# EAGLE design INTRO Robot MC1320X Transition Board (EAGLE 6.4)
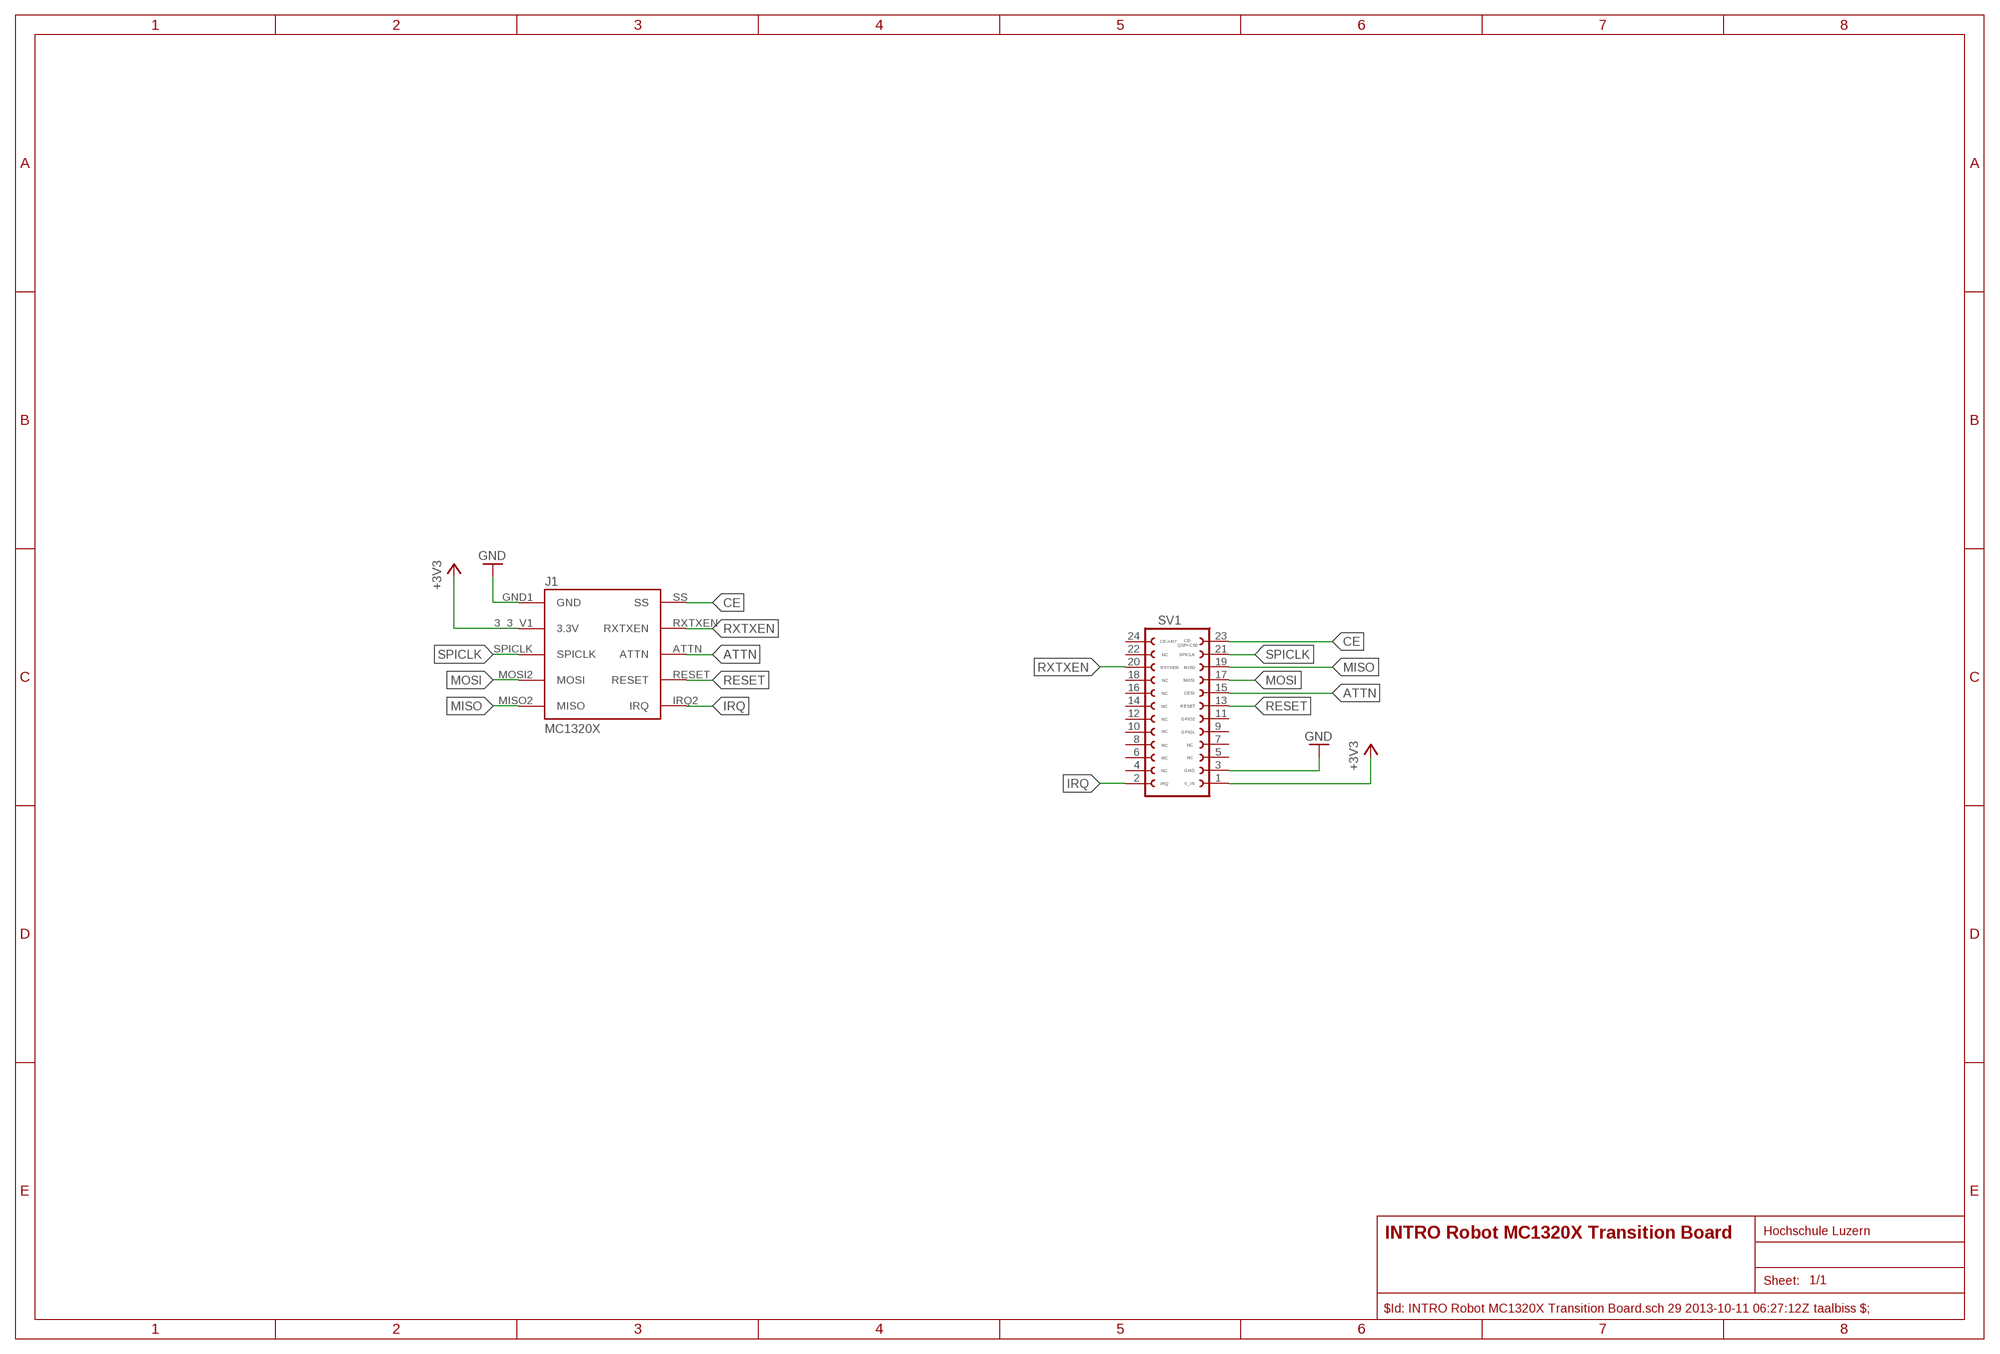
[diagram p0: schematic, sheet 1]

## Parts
J1  MC1320X  MC1320X_MOTHERBOARD  [MC1320X_MOTHERBOARD]
SV1  MC1320X  [FE12-2]

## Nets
+3V3: J1.3_3_V1(3.3V) SV1.1
ATTN: J1.ATTN SV1.15
CE: J1.SS SV1.23
GND: J1.GND1(GND) SV1.3
IRQ: J1.IRQ2(IRQ) SV1.2
MISO: J1.MISO2(MISO) SV1.19
MOSI: J1.MOSI2(MOSI) SV1.17
RESET: J1.RESET SV1.13
RXTXEN: J1.RXTXEN SV1.20
SPICLK: J1.SPICLK SV1.21
Unconnected: SV1.4 SV1.5 SV1.6 SV1.7 SV1.8 SV1.9 SV1.10 SV1.11 SV1.12 SV1.14 SV1.16 SV1.18 SV1.22 SV1.24

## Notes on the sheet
- $Id: INTRO Robot MC1320X Transition Board.sch 29 2013-10-11 06:27:12Z taalbiss $;

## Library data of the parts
J1 = MC1320X_Header_Motherboard:MC1320X_MOTHERBOARD
SV1 = Freescale MC1320x:MC1320X: Freescale MC1320x RF Daughter Board Connector

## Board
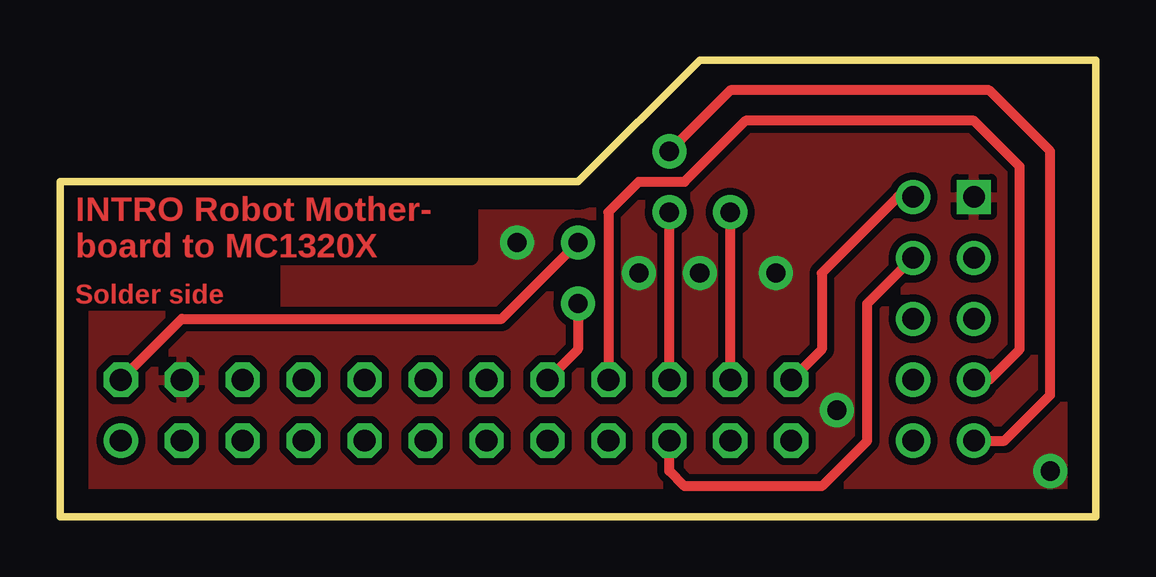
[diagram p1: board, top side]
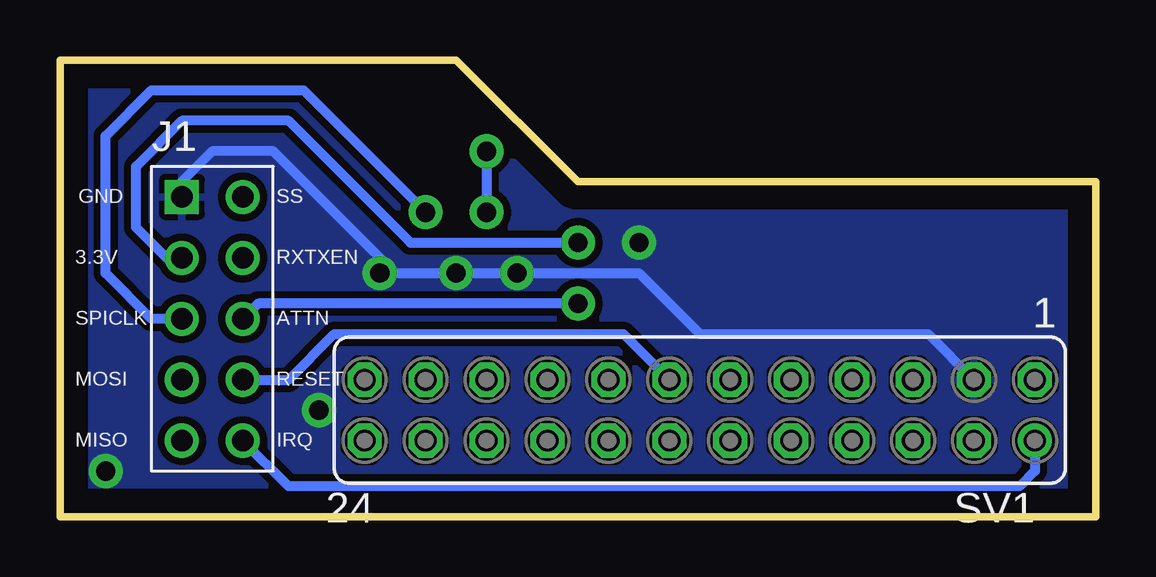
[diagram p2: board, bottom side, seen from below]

Size 43.18 x 19.05 mm. Coordinates in mm from the lower left corner, seen from the top.
Outline: 0,0 43.18,0 43.18,19.05 26.67,19.05 21.59,13.97 0,13.97 0,0
Copper layers (1*16): Top 0.035mm / dielectric 1.5mm / Bottom 0.035mm
Design rules "default": minimum track width 10mil, minimum drill 24mil, track to track 8mil, track to pad 8mil, pad to pad 8mil, via to via 8mil, smd to smd 8mil, copper to edge 40mil, drill to drill 8mil, minimum pad ring 10mil, minimum via ring 8mil, stop-mask expansion 4mil, vias tented up to drill 0mil, thermal gap 10mil
tRestrict: area 0,8.9 to 8.9,14; area 8.9,10.8 to 17.1,14

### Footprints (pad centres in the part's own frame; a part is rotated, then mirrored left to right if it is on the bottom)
MC1320X_MOTHERBOARD = drill 0.9 pad 1.422: 3_3_V1 -1.27,3.81; ATTN 1.27,1.27; IRQ2 1.27,-3.81; MISO2 -1.27,-3.81; MOSI2 -1.27,-1.27; RESET 1.27,-1.27; RXTXEN 1.27,3.81; SPICLK -1.27,1.27; SS 1.27,6.35 | drill 0.9 pad 1.422 square: GND1 -1.27,6.35
FE12-2 = drill 0.914 octagon: 1 -13.97,-1.27; 3 -11.43,-1.27; 4 -11.43,1.27; 5 -8.89,-1.27; 6 -8.89,1.27; 7 -6.35,-1.27; 8 -6.35,1.27; 9 -3.81,-1.27; 10 -3.81,1.27; 11 -1.27,-1.27; 12 -1.27,1.27; 13 1.27,-1.27; 14 1.27,1.27; 15 3.81,-1.27; 16 3.81,1.27; 17 6.35,-1.27; 18 6.35,1.27; 19 8.89,-1.27; 20 8.89,1.27; 21 11.43,-1.27; 22 11.43,1.27; 23 13.97,-1.27; 24 13.97,1.27 | drill 0.914: 2 -13.97,1.27

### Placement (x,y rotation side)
J1  36.83,6.99 0 bottom
SV1  16.51,4.45 180 bottom

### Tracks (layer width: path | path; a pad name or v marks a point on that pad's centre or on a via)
+3V3  (via drill 0.8 pad 1.42)
  Top 0.406: SV1.1 5.08,8.26 18.41,8.26 v21.59,11.43
  Bottom 0.406: J1.3_3_V1 38.73,10.79 40.01,12.06 40.01,14.61 38.1,16.51 33.66,16.51 28.57,11.43 v21.59,11.43
ATTN  (via drill 0.8 pad 1.42)
  Top 0.406: v21.59,8.89 21.59,6.99 SV1.15
  Bottom 0.406: v21.59,8.89 34.92,8.89 J1.ATTN
CE
  Top 0.406: J1.SS 34.92,13.34 31.75,10.16 31.75,6.99 SV1.23
GND  (via drill 0.8 pad 1.42)
  Bottom 0.406: J1.GND1 38.1,13.97 36.83,15.24 34.29,15.24 29.21,10.16 19.05,10.16 16.51,7.62 6.99,7.62 SV1.3
  other vias: 29.84,10.16 24.13,10.16 26.67,10.16 19.05,11.43 41.27,1.91 32.38,4.45
  pour Bottom (isolate 0.305): 0,0 0,13.97 21.59,13.97 26.67,19.05 43.18,19.05 43.18,0
  pour Top (isolate 0.305): 0,0 0,13.97 21.59,13.97 26.67,19.05 43.18,19.05 43.18,0
IRQ
  Bottom 0.406: SV1.2 2.54,1.91 3.17,1.27 33.66,1.27 J1.IRQ2
MISO  (via drill 0.8 pad 1.42)
  Top 0.406: J1.MISO2 39.37,3.17 41.27,5.08 41.27,15.24 38.73,17.78 27.94,17.78 v25.4,15.24 | SV1.19 v25.4,12.7
  Bottom 0.406: v25.4,15.24 v25.4,12.7
MOSI
  Top 0.406: J1.MOSI2 38.73,5.71 40.01,6.99 40.01,14.61 38.1,16.51 28.57,16.51 26.04,13.97 24.13,13.97 22.86,12.7 SV1.17
RESET
  Bottom 0.406: J1.RESET 33.66,5.71 31.75,7.62 19.68,7.62 SV1.13
RXTXEN
  Top 0.406: SV1.20 25.4,1.91 26.04,1.27 31.75,1.27 33.66,3.17 33.66,8.89 J1.RXTXEN
SPICLK  (via drill 0.8 pad 1.42)
  Top 0.406: SV1.21 v27.94,12.7
  Bottom 0.406: J1.SPICLK 39.37,8.26 41.27,10.16 41.27,15.88 39.37,17.78 33.02,17.78 v27.94,12.7

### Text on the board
Top: INTRO Robot Mother- / board to MC1320X | Solder side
